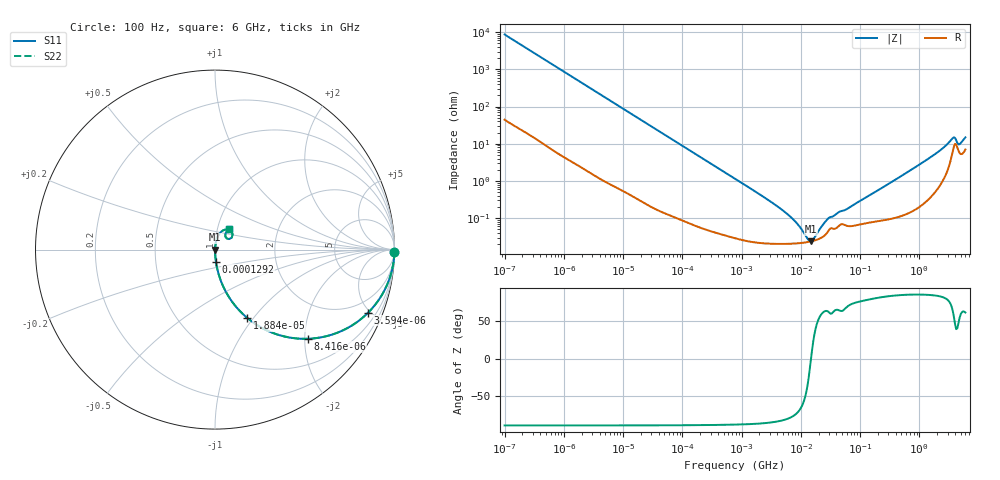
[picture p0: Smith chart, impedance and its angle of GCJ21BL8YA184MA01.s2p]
!Murata Part Number: GCJ21BL8YA184MA01
!These Parameters are Measured in Series Mode Connection
!Data Generated on Mar 13, 2026
!  o--ll--o
!Port1  Port2
!  o------o
!Operation Temp=25[degC], DC Bias Voltage=0[V]
!Freq. Start=100[Hz] Stop=6[GHz] 401[Steps]
# Hz S RI R 50
!Freq.(Hz) S11(Real) S11(Imag) S21(Real) S21(Imag) S12(Real) S12(Imag) S22(Real) S22(Imag)
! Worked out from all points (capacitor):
!   401 points, 100 Hz to 6 GHz, reference 50 ohm
!   read as one part in series: C = 184 nF near 109 Hz
!   lowest |Z| = 23.9 mohm at 14.88 MHz (marker M1)
!   series resonance near 14.88 MHz, so ESL is about 620 pH
!   S11 on the Smith chart (normalised r, x): 100 Hz: open; 3.594 kHz: 1.03, -4.86; 8.416 kHz: 1.01, -2.08; 18.84 kHz: 1.01, -0.93; 129.2 kHz: 1.00, -0.14; 6 GHz: 1.14, +0.26
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100  0.9998 -0.0116  0.000194 0.0116  0.000194 0.0116  0.9998 -0.0116
600  0.9949 -0.0687  0.00509 0.0687  0.00509 0.0687  0.9949 -0.0687
2008  0.9485 -0.2184  0.0515 0.2184  0.0515 0.2184  0.9485 -0.2184
3594  0.8537 -0.3508  0.1463 0.3508  0.1463 0.3508  0.8537 -0.3508
8416  0.5195 -0.4967  0.4805 0.4967  0.4805 0.4967  0.5195 -0.4967
18841  0.18 -0.381  0.82 0.381  0.82 0.381  0.18 -0.381
40335  0.0468 -0.2077  0.9532 0.2077  0.9532 0.2077  0.0468 -0.2077
129199  0.00539 -0.0681  0.9946 0.0681  0.9946 0.0681  0.00539 -0.0681
774597  0.000422 -0.0115  0.9996 0.0115  0.9996 0.0115  0.000422 -0.0115
5554849  0.000206 -0.00139  0.9998 0.00139  0.9998 0.00139  0.000206 -0.00139
8311524  0.000211 -0.000745  0.9998 0.000745  0.9998 0.000745  0.000211 -0.000745
1.300572e7  0.000228 -0.000163  0.9998 0.000163  0.9998 0.000163  0.000228 -0.000163
1.487547e7  0.000238 -2e-07  0.9998 2e-07  0.9998 2e-07  0.000238 -2e-07
1.555665e7  0.000243 5.41e-05  0.9998 -5.41e-05  0.9998 -5.41e-05  0.000243 5.41e-05
2.911731e7  0.000453 0.000881  0.9995 -0.000881  0.9995 -0.000881  0.000453 0.000881
6.233367e7  0.000619 0.00172  0.9994 -0.00172  0.9994 -0.00172  0.000619 0.00172
3.124326e8  0.00101 0.00856  0.999 -0.00856  0.999 -0.00856  0.00101 0.00856
1.712697e9  0.00661 0.0478  0.9934 -0.0478  0.9934 -0.0478  0.00661 0.0478
3.505958e9  0.0561 0.1112  0.9439 -0.1112  0.9439 -0.1112  0.0561 0.1112
3.8344e9  0.0885 0.104  0.9115 -0.104  0.9115 -0.104  0.0885 0.104
4.796499e9  0.0586 0.0709  0.9414 -0.0709  0.9414 -0.0709  0.0586 0.0709
6e9  0.0794 0.1125  0.9206 -0.1125  0.9206 -0.1125  0.0794 0.1125
